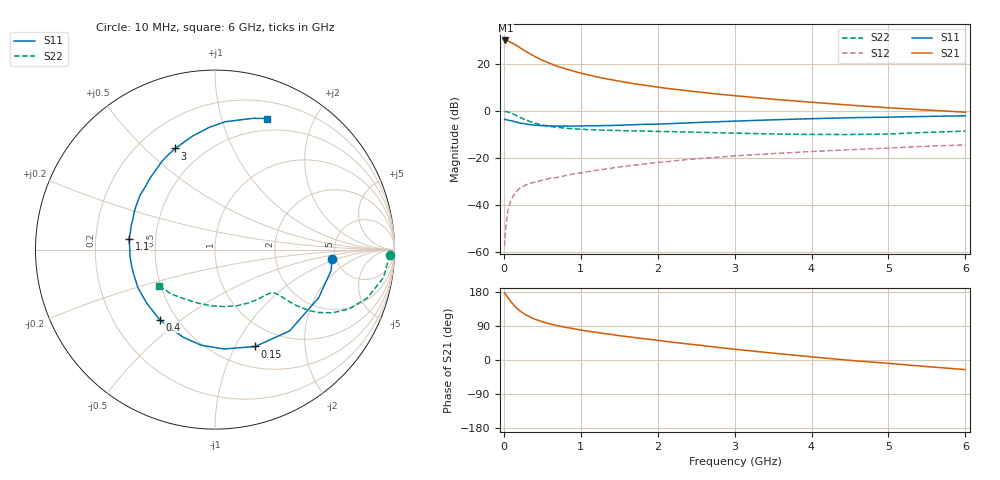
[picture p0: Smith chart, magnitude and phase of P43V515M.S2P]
! SIEMENS Small Signal Semiconductors
! BFP182
! Si NPN RF Bipolar Junction Transistor in SOT143
! VCE = 3.5 V  IC = 15 mA
! Common Emitter S-Parameters:  March  1996
# GHz  S  MA  R  50
!  f  S11  S21  S12  S22
! GHz  MAG  ANG  MAG  ANG  MAG  ANG  MAG  ANG
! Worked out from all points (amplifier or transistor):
!   36 points, 10 MHz to 6 GHz, reference 50 ohm
!   highest |S21| = 30.0 dB at 20 MHz (marker M1)
!   |S21| within 3 dB of that: start of sweep to 205.8 MHz
!   unconditionally stable (mu >= 1): 945.4 MHz to 5.375 GHz
!   at 250 MHz: K = 0.42, MSG = 29.2 dB, |S12| = -32.3 dB
!   at 1.4 GHz: K = 1.12, MAG = 16.7 dB, |S12| = -24.4 dB
!   at 6 GHz: K = 0.92, MSG = 7.0 dB, |S12| = -14.5 dB
!   S11 on the Smith chart (normalised r, x): 10 MHz: 4.59, -0.87; 150 MHz: 0.74, -1.21; 400 MHz: 0.40, -0.42; 1.1 GHz: 0.35, +0.05; 3 GHz: 0.35, +0.62; 6 GHz: 0.37, +1.41
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0.01  0.6531 -4.8  31.65 176.8  0.0013 84.3  0.973 -1.7
0.02  0.6576 -10.1  31.8 174.3  0.0026 86.7  0.9666 -3.7
0.05  0.6369 -24.9  31.12 165.0  0.0073 83.1  0.9522 -9.4
0.1  0.6148 -47.5  28.51 151.8  0.0134 67.7  0.8892 -17.7
0.15  0.5843 -67.5  25.69 140.3  0.018 62.0  0.8166 -23.9
0.2  0.556 -84.7  22.84 131.0  0.022 57.2  0.7424 -28.3
0.25  0.5384 -98.1  20.15 123.5  0.0243 54.0  0.6789 -31.1
0.3  0.5194 -110.0  17.99 117.7  0.027 50.9  0.6269 -32.9
0.4  0.4978 -128.4  14.55 107.9  0.0302 49.2  0.5495 -34.5
0.5  0.4835 -141.9  12.02 100.9  0.0332 48.1  0.4995 -35.1
0.6  0.4794 -153.3  10.32 95.3  0.0365 48.0  0.4665 -35.2
0.7  0.4738 -161.6  8.896 90.6  0.0383 48.9  0.4444 -35.4
0.9  0.4748 -175.3  7.087 82.9  0.0449 49.9  0.4146 -35.9
1.1  0.4828 173.1  5.851 75.9  0.0508 50.3  0.3988 -37.3
1.5  0.4943 156.2  4.304 64.3  0.0634 50.2  0.3814 -41.4
1.8  0.5149 144.4  3.585 56.5  0.0725 49.5  0.3715 -45.6
2.2  0.5375 132.4  2.916 46.8  0.0854 47.1  0.36 -52.2
3  0.6054 111.5  2.112 28.5  0.1097 41.2  0.3355 -68.7
3.5  0.6446 101.3  1.775 18.1  0.1227 37.0  0.3217 -80.6
4.5  0.7148 85.4  1.326 -1.0  0.1489 28.9  0.3129 -107.6
5.5  0.7621 73.7  1.043 -17.4  0.1769 21.1  0.3473 -134.5
6  0.7858 68.3  0.938 -25.3  0.1881 16.2  0.3716 -147.2
